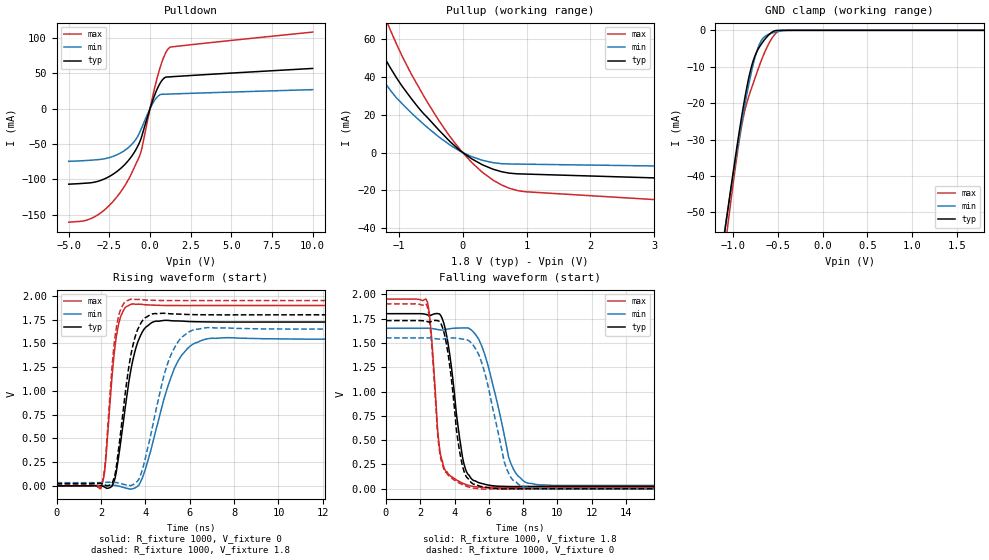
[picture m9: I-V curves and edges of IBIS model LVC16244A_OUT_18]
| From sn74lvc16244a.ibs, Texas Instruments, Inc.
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[Model]   LVC16244A_OUT_18
Model_type  3-state
Enable   Active-Low
Vref =   0
Rref =   1000
Cref =   30p
Vmeas =   0.9
| variable   typ   min   max
C_comp   5.05pF   4.64pF   6.06pF
| C_pullup   8.51pF   3.38pF   19.85pF
| C_pulldown   8.29pF   5.63pF   10.77pF
| C_tri-state   5.05pF   4.64pF   6.06pF
[Temperature Range]   40   100   -40
| Ambient temperature   25   85   -40
[Voltage range]   1.8   1.65   1.95
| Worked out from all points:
|   slope of the pulldown table from 0 to 0.27 V, typ, clamps not added: 14.8 ohm
|   slope of the pullup table from 0 to 0.27 V, typ, clamps not added: 46.7 ohm
|   GND clamp passes 1 mA (typ) near -0.59 V on its own axis
|   rising waveform, R_fixture 1000, V_fixture 0: 20-80 % time 674ps typ, 1.14ns min, 411ps max; typ from 0 V to 1.72 V
|   falling waveform, R_fixture 1000, V_fixture 1.8: 20-80 % time 752ps typ, 1.26ns min, 483ps max; typ from 1.8 V to 0.024 V
|   rising waveform, R_fixture 1000, V_fixture 1.8: 20-80 % time 616ps typ, 1ns min, 389ps max; typ from 0.024 V to 1.8 V
|   falling waveform, R_fixture 1000, V_fixture 0: 20-80 % time 710ps typ, 1.18ns min, 480ps max; typ from 1.73 V to 0 V
[GND Clamp]
| LVC16244A_OUT_18
|   Voltage   I(typ)   I(min)   I(max)
-5V       -855.7mA   -797.6mA   -953.2mA
-1.085V   -53.47mA   -53.15mA   -58.22mA
-1.06V    -49.06mA   -49.09mA   -53.29mA
-975mV    -34.56mA   -35.69mA   -37.29mA
-910mV    -24.24mA   -26.03mA   -26.76mA
-865mV    -17.79mA   -19.78mA   -21.4mA
-800mV    -10.27mA   -11.72mA   -16.17mA
-740mV    -6.037mA   -5.97mA    -11.9mA
-685mV    -3.711mA   -2.772mA   -8.196mA
-590mV    -945.4uA   -940.9uA   -3.072mA
-510mV    -31.84uA   -379.7uA   -498.3uA
1.8V      7.563pA    17.53nA    3.673pA
[Pulldown]
| LVC16244A_OUT_18
|   Voltage   I(typ)   I(min)   I(max)
-5V       -106.8mA   -74.48mA   -160.5mA
-3.945V   -105.3mA   -73.35mA   -157.9mA
-3.11V    -102mA     -71.9mA    -148.6mA
-2.21V    -91.71mA   -66.9mA    -129.5mA
-1.4V     -75.15mA   -56.3mA    -103.1mA
-920mV    -59.95mA   -44.93mA   -80.72mA
-585mV    -44.32mA   -30.88mA   -63.04mA
60mV      4.341mA    2.845mA    6.529mA
455mV     28.54mA    16.86mA    44.89mA
845mV     42.74mA    20.36mA    72.96mA
1.185V    44.91mA    20.64mA    86.07mA
10V       56.83mA    26.86mA    108.2mA
[Pullup]
| LVC16244A_OUT_18
|   Voltage   I(typ)   I(min)   I(max)
-5V       29.31mA    10.34mA    78.9mA
-3.56V    38.96mA    11.4mA     214.8mA
-3.24V    48.87mA    12.22mA    244.5mA
-3.11V    69.83mA    12.77mA    236.3mA
-2.795V   142.2mA    15.56mA    212.5mA
-2.62V    134.9mA    22.74mA    198mA
-2.515V   129.6mA    70.32mA    189mA
-1.885V   92.49mA    69.08mA    132.8mA
-1.13V    44.7mA     32.87mA    64.59mA
-35mV     915.1uA    617uA      1.397mA
860mV     -11.22mA   -6.065mA   -20.08mA
10V       -20.36mA   -10.29mA   -39.14mA
[Ramp]
| LVC16244A_OUT_18
| variable   typ   min   max
dV/dt_r   1.06/7.01E-10   0.95/1.19E-09   1.17/4.31E-10
dV/dt_f   1.07/7.67E-10   0.97/1.33E-09   1.16/5.33E-10
R_load = 1000
[Rising Waveform]
| LVC16244A_OUT_18
R_fixture =   1000
C_fixture =   0
L_fixture =   0
V_fixture =   0
V_fixture_min = 0
V_fixture_max = 0
|   Time   V(typ)   V(min)   V(max)
0s        123.9pV    5.436nV    5.688nV
2.005ns   1.357mV    1.634mV    -20.58mV
2.185ns   -14.92mV   3.579mV    191.6mV
2.525ns   8.027mV    5.339mV    1.217V
2.72ns    186mV      2.059mV    1.607V
3.405ns   1.286V     -32.08mV   1.913V
4.02ns    1.669V     189.5mV    1.906V
5.42ns    1.736V     1.289V     1.898V
6.86ns    1.725V     1.55V      1.898V
50ns      1.724V     1.544V     1.898V
[Falling Waveform]
| LVC16244A_OUT_18
R_fixture =   1000
C_fixture =   0
L_fixture =   0
V_fixture =   1.8
V_fixture_min = 1.65
V_fixture_max = 1.95
|   Time   V(typ)   V(min)   V(max)
0s        1.8V       1.65V      1.95V
2.41ns    1.788V     1.65V      1.923V
3.225ns   1.771V     1.632V     318.3mV
3.67ns    1.438V     1.644V     146.7mV
4.47ns    318.5mV    1.653V     57.66mV
4.94ns    112.9mV    1.637V     29.87mV
5.855ns   42.59mV    1.327V     14.48mV
7.23ns    23.29mV    285.9mV    17.62mV
8.315ns   24.45mV    56.22mV    17.62mV
50ns      24.31mV    33.75mV    17.61mV
[Rising Waveform]
| LVC16244A_OUT_18
R_fixture =   1000
C_fixture =   0
L_fixture =   0
V_fixture =   1.8
V_fixture_min = 1.65
V_fixture_max = 1.95
|   Time   V(typ)   V(min)   V(max)
0s        24.28mV    33.65mV    17.59mV
2.005ns   25.27mV    35.18mV    -1.397mV
2.18ns    10.27mV    36.83mV    211.9mV
2.5ns     27.22mV    38.01mV    1.249V
2.7ns     211.4mV    35.2mV     1.672V
3.375ns   1.408V     5.494mV    1.965V
3.95ns    1.761V     240.5mV    1.957V
5.185ns   1.81V      1.394V     1.95V
6.63ns    1.8V       1.661V     1.95V
50ns      1.8V       1.65V      1.95V
[Falling Waveform]
| LVC16244A_OUT_18
R_fixture =   1000
C_fixture =   0
L_fixture =   0
V_fixture =   0
V_fixture_min = 0
V_fixture_max = 0
|   Time   V(typ)   V(min)   V(max)
0s        1.729V     1.551V     1.901V
2.4ns     1.72V      1.551V     1.878V
3.2ns     1.699V     1.538V     309mV
3.635ns   1.371V     1.549V     138.6mV
4.365ns   316.4mV    1.542V     50.81mV
4.975ns   63.66mV    1.499V     11.76mV
5.73ns    18.74mV    1.211V     -3.368mV
7.005ns   -842.7uV   221.7mV    -602.4uV
8.07ns    -31.28uV   15.84mV    59.48uV
50ns      37.31uV    90.1uV     14.11uV
